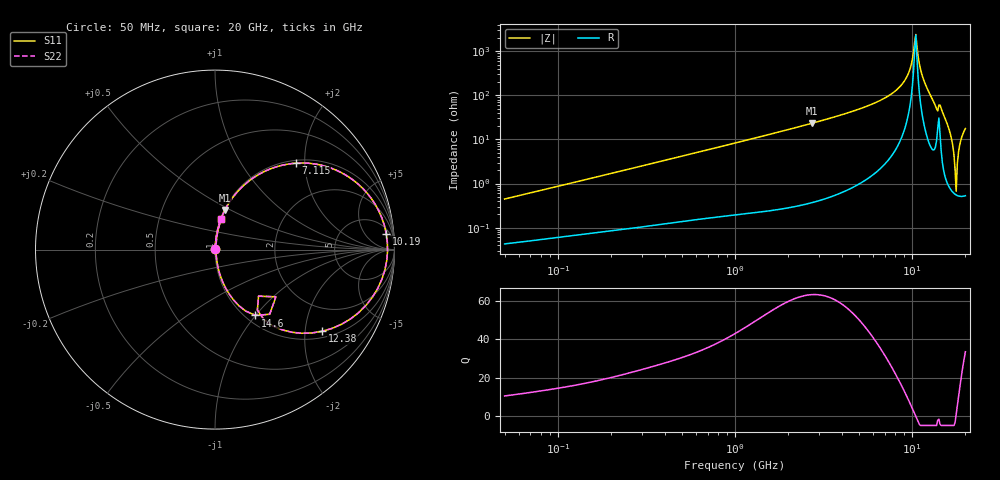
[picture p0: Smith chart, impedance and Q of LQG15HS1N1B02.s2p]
!Murata Part Number: LQG15HS1N1B02
!These Parameters are Measured in Series Mode Connection
!  o--[Z]--o
!Port1  Port2
!  o-------o
!Freq. Start=50[MHz] Stop=20[GHz], 401[Steps]
# Hz S RI R 50
!Freq.(Hz) S11(Real) S11(Imag) S21(Real) S21(Imag) S12(Real) S12(Imag) S22(Real) S22(Imag)
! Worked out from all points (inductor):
!   401 points, 50 MHz to 20 GHz, reference 50 ohm
!   read as one part in series: L = 1.4 nH near 51.52 MHz
!   highest Q = 63.3 at 2.728 GHz (marker M1), where L = 1.37 nH
!   self-resonance near 10.35 GHz
!   S11 on the Smith chart (normalised r, x): 50 MHz: 1.00, +0.01; 7.115 GHz: 1.06, +1.80; 10.19 GHz: 8, +18; 12.38 GHz: 1.18, -2.46; 14.6 GHz: 1.11, -1.00; 20 GHz: 1.01, +0.35
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5e7  0.000446 0.00443  0.9996 -0.00443  0.9996 -0.00443  0.000446 0.00443
1.364002e8  0.000838 0.0117  0.9992 -0.0117  0.9992 -0.0117  0.000838 0.0117
3.721004e8  0.00214 0.0311  0.9979 -0.0311  0.9979 -0.0311  0.00214 0.0311
1e9  0.00873 0.0821  0.9913 -0.0821  0.9913 -0.0821  0.00873 0.0821
2.728004e9  0.0551 0.2204  0.9449 -0.2204  0.9449 -0.2204  0.0551 0.2204
4.89267e9  0.1873 0.3805  0.8127 -0.3805  0.8127 -0.3805  0.1873 0.3805
7.114996e9  0.4503 0.4815  0.5497 -0.4815  0.5497 -0.4815  0.4503 0.4815
7.442007e9  0.5033 0.4822  0.4967 -0.4822  0.4967 -0.4822  0.5033 0.4822
9.178299e9  0.8245 0.3398  0.1755 -0.3398  0.1755 -0.3398  0.8245 0.3398
9.745021e9  0.9126 0.2156  0.0874 -0.2156  0.0874 -0.2156  0.9126 0.2156
1.019291e10  0.9541 0.0888  0.0459 -0.0888  0.0459 -0.0888  0.9541 0.0888
1.066139e10  0.9569 -0.0607  0.0431 0.0607  0.0431 0.0607  0.9569 -0.0607
1.131968e10  0.8774 -0.2646  0.1226 0.2646  0.1226 0.2646  0.8774 -0.2646
1.238412e10  0.596 -0.4555  0.404 0.4555  0.404 0.4555  0.596 -0.4555
1.354865e10  0.2737 -0.3907  0.7263 0.3907  0.7263 0.3907  0.2737 -0.3907
1.460232e10  0.2252 -0.3666  0.7748 0.3666  0.7748 0.3666  0.2252 -0.3666
1.621653e10  0.0335 -0.1565  0.9665 0.1565  0.9665 0.1565  0.0335 -0.1565
1.721783e10  0.00814 -0.0461  0.9919 0.0461  0.9919 0.0461  0.00814 -0.0461
1.774144e10  0.00549 0.00377  0.9945 -0.00377  0.9945 -0.00377  0.00549 0.00377
1.828096e10  0.00773 0.0502  0.9923 -0.0502  0.9923 -0.0502  0.00773 0.0502
1.88369e10  0.0139 0.0932  0.9861 -0.0932  0.9861 -0.0932  0.0139 0.0932
2e10  0.0352 0.1699  0.9648 -0.1699  0.9648 -0.1699  0.0352 0.1699
